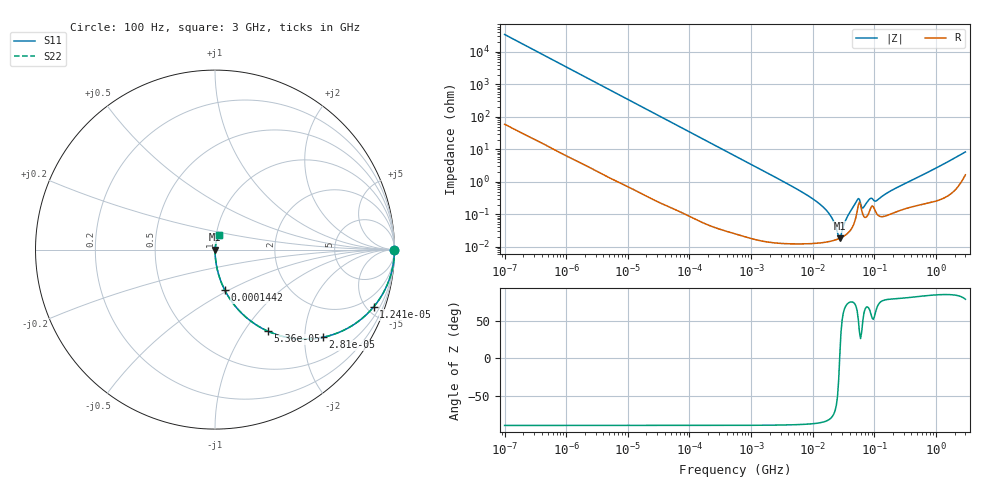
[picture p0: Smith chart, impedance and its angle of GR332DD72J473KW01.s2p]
!Murata Part Number: GR332DD72J473KW01
!These Parameters are Measured in Series Mode Connection
!Data Generated on Mar 13, 2026
!  o--ll--o
!Port1  Port2
!  o------o
!Operation Temp=25[degC], DC Bias Voltage=0[V]
!Freq. Start=100[Hz] Stop=3[GHz] 401[Steps]
# Hz S RI R 50
!Freq.(Hz) S11(Real) S11(Imag) S21(Real) S21(Imag) S12(Real) S12(Imag) S22(Real) S22(Imag)
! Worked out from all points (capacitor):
!   401 points, 100 Hz to 3 GHz, reference 50 ohm
!   read as one part in series: C = 46.5 nF near 109 Hz
!   lowest |Z| = 18.5 mohm at 27.52 MHz (marker M1)
!   series resonance near 27.37 MHz, so ESL is about 730 pH
!   S11 on the Smith chart (normalised r, x): 100 Hz: open; 12.4 kHz: 1.01, -5.55; 28.1 kHz: 1.01, -2.45; 53.6 kHz: 1.00, -1.29; 144.2 kHz: 1.00, -0.48; 3 GHz: 1.03, +0.16
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100  1 -0.00292  1.36e-05 0.00292  1.36e-05 0.00292  1 -0.00292
1788  0.9972 -0.0519  0.00281 0.0519  0.00281 0.0519  0.9972 -0.0519
5024  0.9788 -0.143  0.0212 0.143  0.0212 0.143  0.9788 -0.143
12405  0.8845 -0.3186  0.1155 0.3186  0.1155 0.3186  0.8845 -0.3186
28103  0.6002 -0.4888  0.3998 0.4888  0.3998 0.4888  0.6002 -0.4888
31977  0.5371 -0.4975  0.4629 0.4975  0.4629 0.4975  0.5371 -0.4975
53598  0.2931 -0.454  0.7069 0.454  0.7069 0.454  0.2931 -0.454
144239  0.0547 -0.2261  0.9453 0.2261  0.9453 0.2261  0.0547 -0.2261
547723  0.00422 -0.0628  0.9958 0.0628  0.9958 0.0628  0.00422 -0.0628
9794414  0.000136 -0.0031  0.9999 0.0031  0.9999 0.0031  0.000136 -0.0031
1.789277e7  0.000146 -0.00113  0.9999 0.00113  0.9999 0.00113  0.000146 -0.00113
2.12544e7  0.000156 -0.000663  0.9998 0.000663  0.9998 0.000663  0.000156 -0.000663
2.52476e7  0.000173 -0.000212  0.9998 0.000212  0.9998 0.000212  0.000173 -0.000212
2.751729e7  0.000185 1.46e-05  0.9998 -1.46e-05  0.9998 -1.46e-05  0.000185 1.46e-05
2.872754e7  0.000192 0.00013  0.9998 -0.00013  0.9998 -0.00013  0.000192 0.00013
3.71925e7  0.000267 0.000876  0.9997 -0.000876  0.9997 -0.000876  0.000267 0.000876
5.248048e7  0.00122 0.00244  0.9988 -0.00244  0.9988 -0.00244  0.00122 0.00244
6.794454e7  0.000847 0.0015  0.9992 -0.0015  0.9992 -0.0015  0.000847 0.0015
8.425944e7  0.00132 0.00269  0.9987 -0.00269  0.9987 -0.00269  0.00132 0.00269
1.090876e8  0.00106 0.00243  0.9989 -0.00243  0.9989 -0.00243  0.00106 0.00243
1.751444e8  0.00101 0.00491  0.999 -0.00491  0.999 -0.00491  0.00101 0.00491
3e9  0.0225 0.0786  0.9775 -0.0786  0.9775 -0.0786  0.0225 0.0786
